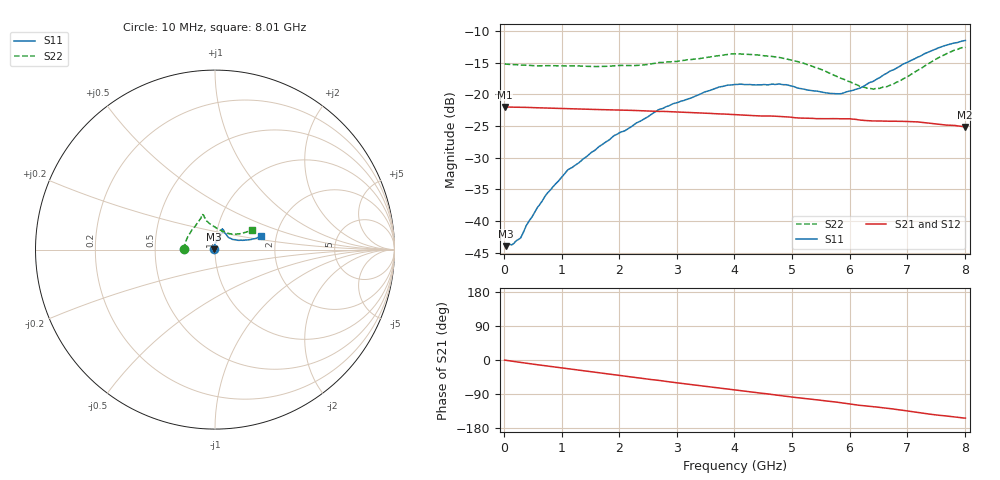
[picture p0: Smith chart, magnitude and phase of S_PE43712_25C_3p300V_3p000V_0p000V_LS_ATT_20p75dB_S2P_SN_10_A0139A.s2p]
! DEVICE ID: PE43712
! File Path: z:\PE43713\PE43713_CHAR_NOM_04292014\AMB\3p300\LS_ATT_20p75dB\PE43713_AMB_3p300V_3p000V_0p000V_LS_ATT_20p75dB_S2P_SN_10_A0139A.s2p
! Serial: 10
! Lot: A0139A
! Temp: 25C
! VDD: 3.300
! VSS: 0.000
! Control_Hi: 3.000
! Control_Lo: 0.000
! Attenuation Step: 20.75dB
! Port 1: RF1
! Port 2: RF2
! ThroughPath:1-2
! IDD: 0.0001467811
! ISS: -1.32e-007
#  Hz  S  RI  R  50
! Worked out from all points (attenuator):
!   801 points, 10 MHz to 8.01 GHz, reference 50 ohm
!   highest |S21| = -21.98 dB at 10 MHz (marker M1); lowest = -25.1 dB at 8 GHz (marker M2)
!   lowest |S11| = -44.0 dB at 30 MHz (marker M3), VSWR 1.01, Z = 49.4 + j0.135 ohm
!   |S11| at or under -10 dB: start of sweep to end of sweep
!   |S22| runs from -19.2 to -12.6 dB; largest |S21 - S12| = 0.00029
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1e7  -0.00657 0.000568  0.0796 -0.000385  0.0796 -0.000378  -0.1738 0.00116
3e7  -0.00619 0.00137  0.0795 -0.000989  0.0796 -0.001  -0.1732 0.00287
1.5e8  -0.00536 0.00376  0.0792 -0.00468  0.0792 -0.00468  -0.1717 0.0107
2.8e8  -0.00456 0.00572  0.0786 -0.00851  0.0787 -0.00854  -0.1698 0.0176
4.2e8  -0.00432 0.00876  0.0779 -0.0126  0.0778 -0.0126  -0.168 0.025
7.4e8  -0.00396 0.0159  0.0751 -0.0213  0.0751 -0.0213  -0.1628 0.0438
1.1e9  -0.00252 0.025  0.0709 -0.0301  0.0709 -0.0302  -0.1553 0.0633
1.35e9  -5.2e-05 0.0303  0.0677 -0.0358  0.0677 -0.0358  -0.1493 0.075
1.91e9  0.00871 0.0464  0.0588 -0.0472  0.0587 -0.0472  -0.1307 0.1059
2.68e9  0.0268 0.0706  0.0434 -0.0591  0.0434 -0.0591  -0.0994 0.1478
3.71e9  0.039 0.1063  0.0197 -0.0674  0.0196 -0.0674  -0.0746 0.1873
4.01e9  0.0402 0.1128  0.0127 -0.0681  0.0127 -0.0681  -0.074 0.1954
4.79e9  0.044 0.1124  -0.00441 -0.0669  -0.00441 -0.0669  -0.0616 0.1853
5.35e9  0.0564 0.0908  -0.0153 -0.0629  -0.0153 -0.0629  -0.047 0.1603
5.87e9  0.0771 0.0665  -0.0251 -0.0591  -0.0251 -0.0591  -0.0117 0.1326
6.17e9  0.0954 0.0578  -0.031 -0.0547  -0.0308 -0.0547  0.0163 0.1149
6.33e9  0.1097 0.0555  -0.0328 -0.0526  -0.0327 -0.0526  0.0348 0.1064
6.68e9  0.1414 0.0519  -0.0377 -0.0484  -0.0376 -0.0484  0.0746 0.0902
7e9  0.1706 0.0533  -0.0427 -0.0437  -0.0426 -0.0436  0.1074 0.0856
7.54e9  0.2243 0.0619  -0.0479 -0.0328  -0.0478 -0.0327  0.1688 0.0961
8e9  0.255 0.0754  -0.0495 -0.0249  -0.0494 -0.025  0.2075 0.1097
8.01e9  0.2555 0.0761  -0.0495 -0.0249  -0.0494 -0.0249  0.2081 0.1098
